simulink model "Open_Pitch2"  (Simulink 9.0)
settings: Solver=ode45  StartTime=0.0  StopTime=150  RelTol=1e-3  EnableMultiTasking=on
InitFcn:
  | r2d= 180/pi; d2r=pi/180;
  | [Ap,Bp,Cp,Dp]= vehi_pitch;                    % Load the Pitch Analysis Model
  | load Kc.mat -ascii
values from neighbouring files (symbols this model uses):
  Cza = -0.032    [init_pitch.m]    (also in init.m)
  Czde = -0.0087    [init_pitch.m]    (also in init.m)
  Mv = 1219.1    [init_pitch.m]    (also in init.m; init_lat.m)
  Qbar = 1220.6    [init_pitch.m]    (also in init.m; init_lat.m)
  Sref = 145.4    [init_pitch.m]    (also in init.m; init_lat.m)
undefined symbols (not defined in the file or in its folder): Ap, Bp, Cp, Dp, Kc

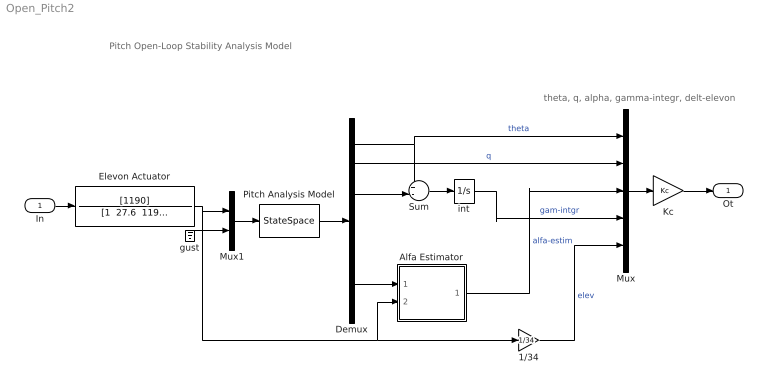
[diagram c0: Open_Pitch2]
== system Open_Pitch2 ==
  note: Pitch Open-Loop Stability Analysis Model
  note: theta, q, alpha, gamma-integr, delt-elevon
  In : Inport
  1/34 : Gain  Gain=1/34
  Alfa Estimator : Subsystem
  Demux : Demux  Outputs=7
  Elevon Actuator : TransferFcn  Numerator=[1190]  Denominator="[1  27.6  1190]"
  Kc : Gain  Gain=Kc  Multiplication=Matrix(K*u)
  Mux : Mux  Inputs=5
  Mux1 : Mux  Inputs=2
  Pitch Analysis Model : StateSpace  A=Ap  B=Bp  C=Cp  D=Dp  InitialCondition=0
  Sum : Sum  Inputs=+-|
  gust : Ground
  int : Integrator
  Ot : Outport
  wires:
  Demux/1 -> Mux/1, Sum/1  "theta"
  Mux/1 -> Kc/1
  1/34/1 -> Mux/5  "elev"
  int/1 -> Mux/4  "gam-intgr"
  Sum/1 -> int/1
  Kc/1 -> Ot/1
  Mux1/1 -> Pitch Analysis Model/1
  In/1 -> Elevon Actuator/1
  gust/1 -> Mux1/2
  Elevon Actuator/1 -> Alfa Estimator/2(d-elev), 1/34/1, Mux1/1
  Pitch Analysis Model/1 -> Demux/1
  Demux/2 -> Mux/2  "q"
  Demux/3 -> Sum/2
  Demux/6 -> Alfa Estimator/1(Nz)
  Alfa Estimator/1(alf_est) -> Mux/3  "alfa-estim"

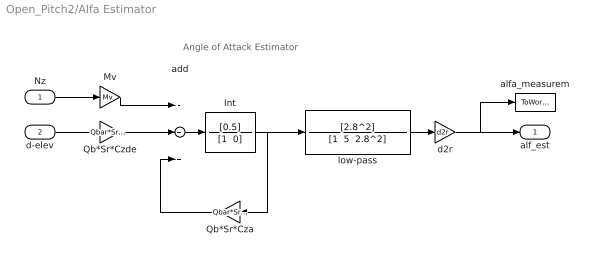
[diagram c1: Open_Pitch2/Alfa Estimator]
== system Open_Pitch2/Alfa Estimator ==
  note: Angle of Attack Estimator
  Nz : Inport
  d-elev : Inport  Port=2
  Int : TransferFcn  Numerator=[0.5]  Denominator="[1  0]"
  Mv : Gain  Gain=Mv
  Qb*Sr*Cza : Gain  Gain=Qbar*Sref*Cza
  Qb*Sr*Czde : Gain  Gain=Qbar*Sref*Czde*r2d
  add : Sum  Inputs=-++
  alfa_measurem : ToWorkspace  VariableName=alfa_est  SampleTime=-1
  d2r : Gain  Gain=d2r
  low-pass : TransferFcn  Numerator=[2.8^2]  Denominator="[1  5  2.8^2]"
  alf_est : Outport
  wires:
  add/1 -> Int/1
  Qb*Sr*Cza/1 -> add/3
  Mv/1 -> add/1
  Qb*Sr*Czde/1 -> add/2
  Int/1 -> Qb*Sr*Cza/1, low-pass/1
  d-elev/1 -> Qb*Sr*Czde/1
  Nz/1 -> Mv/1
  low-pass/1 -> d2r/1
  d2r/1 -> alf_est/1, alfa_measurem/1
